FUNCTION_BLOCK "IMAC_TANK"
TITLE = TANK
//--------------------------------------------------------------------------------
//SIEMENS AG     I&S IP PEP SN                        PSP-Element: D-09300081-E-E5
//--------------------------------------------------------------------------------
//History
//=======
//Date      Version  Description                                   Author
//2004/12/02   1.0   Basic Edition converted to S7                 Edelmann
//
//--------------------------------------------------------------------------------
//PLC:   >= S7-300
//--------------------------------------------------------------------------------
//Specification:   Refer "IMAC_L_TankContents.doc"
//--------------------------------------------------------------------------------
//
//--------------------------------------------------------------------------------
//Called FC: FC166 "GetSts_ex"
//           FC167 "GetValue_ex"
//           FC114 "abvspu_XPO_NORM"
//           SFC20 "BLKMOV"
//--------------------------------------------------------------------------------
//
//--------------------------------------------------------------------------------
//Note:
//Pressure MePo        : ................................... [Bar]
//Level MePo           : ................................... [m]
//Volume               : ................................... [m3]
//Temperature MePo     : ................................... [°C]
//Temperature Setpoint : ................................... [°C]
//Density              : ................................... [kg/dm3]
//Mass                 : ................................... [Tons]
//Vol.-Exp.Coefficient : ................................... [1/K]
//
//--------------------------------------------------------------------------------
// KNOW_HOW_PROTECT
AUTHOR : Edelmann
FAMILY : IMAC
NAME : Tank
VERSION : 1.0


VAR_INPUT
  OBJ : INT ;
  XTsub : REAL  := 2.000000e+001;	//Temperature substitute value from OS [°C]
  XDensity : REAL  := 1.000000e+000;	//Setpoint Density from OS [kg/dm3]
  XRefTemp : REAL ;	//Setpoint Temperature for Density setpoint from OS [°C]
  XVEC : REAL ;	//Volumetric expansion coefficient [1/K]
  PCONF : STRUCT
   LastRecord : INT  := 100;
   Pointer1stRecord : STRUCT
    S7ID : BYTE  := B#16#10;	//ANY pointer: ID S7
    RepeatFactor : INT  := 44;	//ANY pointer: repeat factor
    Typ : BYTE  := B#16#2;	//ANY pointer: data typ =02 BYTE =04 WORD =05 INT =06 DWORD =07 DINT =08 REAL
    DBNo : INT  := 85;	//ANY pointer: DB number, zero if no DB
    MemoryArea : BYTE  := B#16#84;	//ANY pointer: Memory area =81 IN =82 OUT =83 M =84 DB =85 DI =86 L
    DWHigh : BYTE ;	//ANY pointer: DW highest byte
    DWX : INT ;	//ANY pointer: DW low / bit (address = byte *8 + bit)
   END_STRUCT ;
  END_STRUCT ;
END_VAR
VAR_OUTPUT
  YVolume : REAL ;	//Volume [m3]
  YMass : REAL ;	//Mass [Tons]
  YLevel : REAL ;	//Level [m]
  OSSTAT : WORD ;	//Status for OS
  OSALARM : WORD ;	//Alarms for OS
END_VAR
VAR
  Tank : STRUCT
   PCONF : STRUCT
    ObjInput : INT ;	//Objectnumber of pressure/level transmitter
    ObjTemp : INT ;	//Objectnumber of temperature transmitter
    SklRefNo : BYTE ;	//Number of tank table
    Offset : REAL ;	//Offset of pressure transmitter from bottom of tank [m]
    LL_XTsub : REAL  := -5.000000e+001;	//Low limit tank temperature [°C]
    HL_XTsub : REAL  := 5.000000e+001;	//High limit tank temperature [°C]
    LL_XDensity : REAL  := 5.000000e-001;	//Low limit medium density [kg/dm3]
    HL_XDensity : REAL  := 1.500000e+000;	//High limit medium density [kg/dm3]
    LL_XRefTemp : REAL  := -5.000000e+001;	//Low limit reference temperature for density [°C]
    HL_XRefTemp : REAL  := 5.000000e+001;	//High limit reference temperature for density [°C]
    LL_XVEC : REAL ;	//Low limit volume expansion coefficient [1/K]
    HL_XVEC : REAL  := 1.000000e-002;	//High limit volume expansion coefficient [1/K]
    Modeswitches : STRUCT
     M0_SensorConfiguration : BOOL ;	// 0: Pressure Sensor;  1: Level Sensor
     M1_TemperatureComp : BOOL ;	// 0: without Compensation;   1: with compensation
     M2 : BOOL ;	//
     M3 : BOOL ;	//
     M4 : BOOL ;	//
     M5 : BOOL ;	//
     M6 : BOOL ;
     M7 : BOOL ;	//
     M8 : BOOL ;	//
     M9 : BOOL ;	//
     M10 : BOOL ;
     M11 : BOOL ;
     M12 : BOOL ;
     M13 : BOOL ;
     M14 : BOOL ;
     M15 : BOOL ;	//
    END_STRUCT ;
   END_STRUCT ;
  END_STRUCT ;
  siFailRR : INT ;	//Failure blockmove read record
  siFailWR : INT ;	//Failure blockmove write record
END_VAR
VAR_TEMP
  tbResultGetSts : BOOL ;	//Return value read status
  tbResultGetVal : BOOL ;	//Return value read value
  tbMPLevelOOR : BOOL ;	//MePo PRESSURE out of range
  tbMPLevelUndef : BOOL ;	//MePo PRESSURE undefined
  tbMPLevelFadedOut : BOOL ;	//MePo PRESSURE faded out
  tbMPTempFault : BOOL ;	//MePo TEMPERATURE is in fault state
  trXTsub : REAL ;	//Operator setpoint for temperature
  trXDensity : REAL ;	//Operator setpoint for density
  trXRefTemp : REAL ;	//Operator setpoint for reference density temperature
  trXVEC : REAL ;	//Operator setpoint for volume expansion coefficiency
  tiStatusMPLevel : INT ;	//Statusword from MP pressure/level transmitter
  tiStatusMPTemp : INT ;	//Statusword from temperature transmitter
  trMPValueLevel : REAL ;	//Pressure/level value from transmitter
  trMPValueTemp : REAL ;	//Temperature value from transmitter
  trLevel : REAL ;	//Computed level
  trTemperature : REAL ;	//Computed temperature
  trDensity : REAL ;	//Computed density
  trVolume : REAL ;	//Computed volume
  trMass : REAL ;	//Computed mass
  P_currentRecord : ANY ;	//ANY pointer of the current record
END_VAR
BEGIN
NETWORK
TITLE =Calculation of current ANY pointer for reading /writing record
// ANY-pointer of current record
      L     #PCONF.Pointer1stRecord.S7ID;
      T     LB    50;
      L     #PCONF.Pointer1stRecord.Typ;
      T     LB    51;
      L     #PCONF.Pointer1stRecord.RepeatFactor;
      T     LW    52;
      L     #PCONF.Pointer1stRecord.DBNo;
      T     LW    54;
      L     #PCONF.Pointer1stRecord.MemoryArea;
      T     LB    56;
      L     #PCONF.Pointer1stRecord.DWHigh;
      T     LB    57;
      L     #PCONF.Pointer1stRecord.DWX;
      T     LW    58;

      L     #OBJ; //Check whether Obj within the range
      L     #PCONF.LastRecord;
      >I    ;
      SPB   cRcd;
      L     #OBJ;
      L     1;
      <I    ;
      SPB   cRcd;
      L     #OBJ;
cRcd: +     -1;
      L     #PCONF.Pointer1stRecord.RepeatFactor;
      *I    ;
      SLD   3; //DBW + DBX address of the current record
      L     LD    56;
      OD    ;
      T     LD    56; //DBWX part of ANY pointer "P_currentRecord"
NETWORK
TITLE =Read record

      CALL "BLKMOV" (
           SRCBLK                   := #P_currentRecord,
           RET_VAL                  := #siFailRR,
           DSTBLK                   := #Tank);

NETWORK
TITLE =Check operator value inputs
//If value < low limit set value to low limit
//If value > high limit set value to high limit
//
//XTsub
      L     #XTsub; //Read input XTsub
      T     #trXTsub;
      L     #Tank.PCONF.LL_XTsub; //< low level ?
      <R    ;
      SPB   OOR1;

      TAK   ;
      L     #Tank.PCONF.HL_XTsub; //> high level ?
      >R    ;
      SPB   OOR1;
      SPA   DENS;

OOR1: T     #trXTsub;

//XDensity
DENS: L     #XDensity; //Read input XDENSITY
      T     #trXDensity;
      L     #Tank.PCONF.LL_XDensity; //< low level ?
      <R    ;
      SPB   OOR2;

      TAK   ;
      L     #Tank.PCONF.HL_XDensity; //> high level ?
      >R    ;
      SPB   OOR2;
      SPA   TEMP;

OOR2: T     #trXDensity;

//XRefTemp
TEMP: L     #XRefTemp; //Read input XRefTemp
      T     #trXRefTemp;
      L     #Tank.PCONF.LL_XRefTemp; //< low level ?
      <R    ;
      SPB   OOR3;

      TAK   ;
      L     #Tank.PCONF.HL_XRefTemp; //> high level ?
      >R    ;
      SPB   OOR3;
      SPA   XVEC;

OOR3: T     #trXRefTemp;

//XVEC
XVEC: L     #XVEC; //Read input XVEC
      T     #trXVEC;
      L     #Tank.PCONF.LL_XVEC; //< low level ?
      <R    ;
      SPB   OOR4;

      TAK   ;
      L     #Tank.PCONF.HL_XVEC; //> high level ?
      >R    ;
      SPB   OOR4;
      SPA   ENDC;

OOR4: T     #trXVEC;
ENDC: NOP   0;
NETWORK
TITLE =Read Input (Pressure/Level) from external object
// Get status of the analogue MePo for tank level
      CALL "GetSts_ex" (
           obj                      := #Tank.PCONF.ObjInput,//Objectnumber of analogue value
           wMask                    := W#16#1F,// Bit Mask for Significant Bits of Status (Bits 0-4)
           wSts                     := #tiStatusMPLevel,// Status as a return Value
           bOk                      := #tbResultGetSts);// Result Flag of FC166:GetSts_ex

// Get value of the analogue MePo for tank level
      CALL "GetValue_ex" (
           obj                      := #Tank.PCONF.ObjInput,//Objectnumber of analogue value
           iVal                     := LD    70,//Dummy
           rVal                     := #trMPValueLevel,//Value (Real) of MePo for pressure/level
           bVal                     := L     70.0,//Dummy
           bOk                      := #tbResultGetVal);//Result flag of FC167:GetVal_ex

// Compute the 'Fault' Flag for tank level
      L     #tiStatusMPLevel; // Status as a return Value
      L     16; // AbvSPU Status 'Out of Range'
      ==I   ; // Out of Range ?
      =     #tbMPLevelOOR;

      TAK   ;
      L     17; // AbvSPU Status 'Undefinded'
      ==I   ; // Undefined ?
      ON    #tbResultGetSts; // Fault in 'GetSts_ex' ?
      ON    #tbResultGetVal; // Fault in 'GetVal_ex' ?
      =     #tbMPLevelUndef;

      TAK   ;
      L     18; // AbvSPU Status 'Faded Out'
      ==I   ; // Faded Out ?
      =     #tbMPLevelFadedOut;
NETWORK
TITLE =Read Input (temperature) from external object
// Get status of the analogue MePo for tank temperature
      CALL "GetSts_ex" (
           obj                      := #Tank.PCONF.ObjTemp,//Objectnumber of analogue value
           wMask                    := W#16#1F,// Bit Mask for Significant Bits of Status (Bits 0-4)
           wSts                     := #tiStatusMPTemp,// Status as a return Value
           bOk                      := #tbResultGetSts);// Result Flag of FC166:GetSts_ex

// Get value of the analogue MePo for tank temperature
      CALL "GetValue_ex" (
           obj                      := #Tank.PCONF.ObjTemp,//Objectnumber of analogue value
           iVal                     := LD    70,//Dummy
           rVal                     := #trMPValueTemp,//Value (Real) of MePo for temperature
           bVal                     := L     70.0,//Dummy
           bOk                      := #tbResultGetVal);//Result flag of FC167:GetVal_ex

// Compute the 'Fault' Flag for tank temperature
      ON    #tbResultGetSts; // Fault in 'GetSts_ex' ?
      ON    #tbResultGetVal; // Fault in 'GetVal_ex' ?
      O(    ;
      L     #tiStatusMPTemp; // Status as a return Value
      L     16; // AbvSPU Status 'Out of Range'
      ==I   ; // Out of Range ?
      )     ;
      O(    ;
      TAK   ;
      L     17; // AbvSPU Status 'Undefinded'
      ==I   ; // Undefined ?
      )     ;
      O(    ;
      TAK   ;
      L     18; // AbvSPU Status 'Faded Out'
      ==I   ; // Faded Out ?
      )     ;
      =     #tbMPTempFault; // Fault of the temperature MePo

NETWORK
TITLE =Compute tank temperature
//If temperature from extern MP object is available then use it.
//Otherwise use OS setpoint temperature value.
//
      U     #tbMPTempFault; //Temperature MP useable?
      SPB   OS;
      L     #trMPValueTemp; //Read MP Temperature value
      SPA   ENDT;

OS:   L     #trXTsub; //Read OS temperature setpoint

ENDT: T     #trTemperature;
NETWORK
TITLE =Compute actual density
//If volumetric expansion coefficient is engineered (<>0) the density is computed
//as following term:
//
//                                      Density (t ref)
//Density(act) = ------------------------------------------------------------
//                  1 + [Volumetric expansion coefficient * (t act - t ref)]
//
//If a compute density is not available set density to density (t ref)
      L     #trXVEC; //Read volumetric expansion coefficient from input
      L     0; //volumetric expansion coefficien engineered
      ==R   ;
      ON    #Tank.PCONF.Modeswitches.M1_TemperatureComp; //Temperature compensation switched off?
      SPB   NOAV;

      L     #trTemperature; //tank temperature
      L     #trXRefTemp; //Reference temperature (t ref) to density (t ref)
      -R    ;
      L     #trXVEC; //Volumetric expansion coefficient
      *R    ;
      L     1.000000e+000;
      +R    ;
      L     #trXDensity; //Density (t ref)
      TAK   ;
      /R    ; //Density(t ref)/[1+(VEC *(temp-temp ref))]
      SPA   ENDD;

NOAV: L     #trXDensity; //Read density (t ref)

ENDD: T     #trDensity;
NETWORK
TITLE =Compute real tank level
//If the input signal is a level value
//(Tank.PCONF.Modeswitches.M0_SensorConfiguration = 1) then the input value is
//already the tank level.
//
//If the input signal is a pressure value
//(Tank.PCONF.Modeswitches.M0_SensorConfiguration = 0) then the level has to be
//calculated as following term:
//
//                    pressure [bar] * 100
//level [m] = ------------------------------------ + offset (sensor) [m]
//              density[kg/dm3] * gravity[m/s2]
//
      U     #Tank.PCONF.Modeswitches.M0_SensorConfiguration; //Level transmitter ?
      SPB   LT;

      L     #trDensity; //computed Density
      L     9.810000e+000; //Gravity
      *R    ;
      L     #trMPValueLevel; //Read value from pressure transmitter
      TAK   ;
      /R    ;
      L     1.000000e+002;
      *R    ;
      L     #Tank.PCONF.Offset; //Offset of transmitter from tank bottom
      +R    ; //(pressure/(density*gravity))+offset
      SPA   ENDL;

LT:   L     #trMPValueLevel; //Read value from level transmitter

ENDL: T     #trLevel; //Real tank level
NETWORK
TITLE =Get corresponding volume via tank table
//Scalegroups in DB188
      CALL "abvspu_XPO_NORM" (
           PODX                     := #Tank.PCONF.SklRefNo,//Tank table number
           ROHW                     := #trLevel,//Tank level
           NRMV                     := #trVolume);//Computed volume

NETWORK
TITLE =Compute mass
//mass = volume * density
      L     #trVolume; //Read volume
      L     #trDensity; //Read density
      *R    ;
      T     #trMass; //Store to mass

NETWORK
TITLE =Outputs
//hold last valid value in output in case of input failure
      O     #tbMPLevelOOR; //Input value out of range?
      O     #tbMPLevelUndef; //Input value undefined?
      O     #tbMPLevelFadedOut; //Input value Faded out?
      SPB   EOUT;

      L     #trVolume; //Read volume
      T     #YVolume; //Store to output
      L     #trMass; //Read mass
      T     #YMass; //Store to output
      L     #trLevel; //Read level
      T     #YLevel; //Store to output

EOUT: NOP   0; //No change because input is not valid (hold last valid outputs)
NETWORK
TITLE =Statusword
//Transfer statusword of volume/level value to OSSTAT.
//In case of input failure set status to "undefined"
      L     #tiStatusMPLevel; //Statusword of volume/level value
      T     #OSSTAT; //to output

      U     #tbResultGetSts; //No fault in 'GetSts_ex' ?
      U     #tbResultGetVal; //No fault in 'GetVal_ex' ?
      SPB   ESTA;
      L     17; //State: Undefined
      T     #OSSTAT; //to output

ESTA: NOP   0;
NETWORK
TITLE =Write record

      CALL "BLKMOV" (
           SRCBLK                   := #Tank,
           RET_VAL                  := #siFailWR,
           DSTBLK                   := #P_currentRecord);

END_FUNCTION_BLOCK

